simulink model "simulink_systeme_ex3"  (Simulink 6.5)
settings: Solver=ode45  StartTime=0.0  StopTime=.2  RelTol=1e-3
PostLoadFcn:
  | simulink_systems_ex3
InitFcn:
  | simulink_systems_ex3
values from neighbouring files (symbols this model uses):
  A = [-2*D*w -w^2 ; 1 0]    [simulink_systems_ex3.m]
  B = [w^2 ; 0 ]    [simulink_systems_ex3.m]
  C = [0 1]    [simulink_systems_ex3.m]
  D = 0    [simulink_systems_ex3.m]

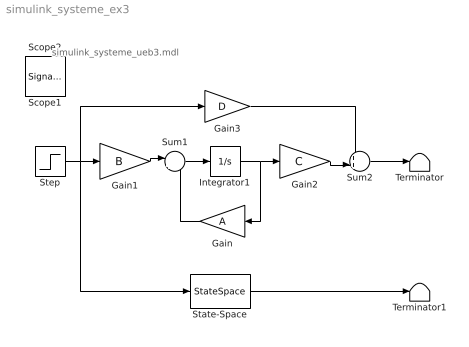
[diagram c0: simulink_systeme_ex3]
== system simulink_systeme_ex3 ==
  note: simulink_systeme_ueb3.mdl
  Gain : Gain  Orientation=left  Gain=A  Multiplication=Matrix(K*u)
  Gain1 : Gain  Gain=B  Multiplication=Matrix(K*u)
  Gain2 : Gain  Gain=C  Multiplication=Matrix(K*u)
  Gain3 : Gain  Gain=D  Multiplication=Matrix(K*u)
  Integrator1 : Integrator
  State-Space : StateSpace  A=A  B=B  C=C  D=D
  Step : Step  Time=.1  SampleTime=0
  Sum1 : Sum  Inputs=|++
  Sum2 : Sum  Inputs=++|
  Terminator : Terminator
  Terminator1 : Terminator
  Scope1 : SignalViewerScope  IOType=viewer  RefreshTime=0.035000
  Scope2 : SignalViewerScope  IOType=viewer  RefreshTime=0.035000
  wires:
  Step/1 -> Gain3/1, Gain1/1, State-Space/1
  State-Space/1 -> Terminator1/1
  Sum1/1 -> Integrator1/1
  Integrator1/1 -> Gain2/1, Gain/1
  Gain/1 -> Sum1/2
  Gain1/1 -> Sum1/1
  Gain3/1 -> Sum2/1
  Gain2/1 -> Sum2/2
  Sum2/1 -> Terminator/1
